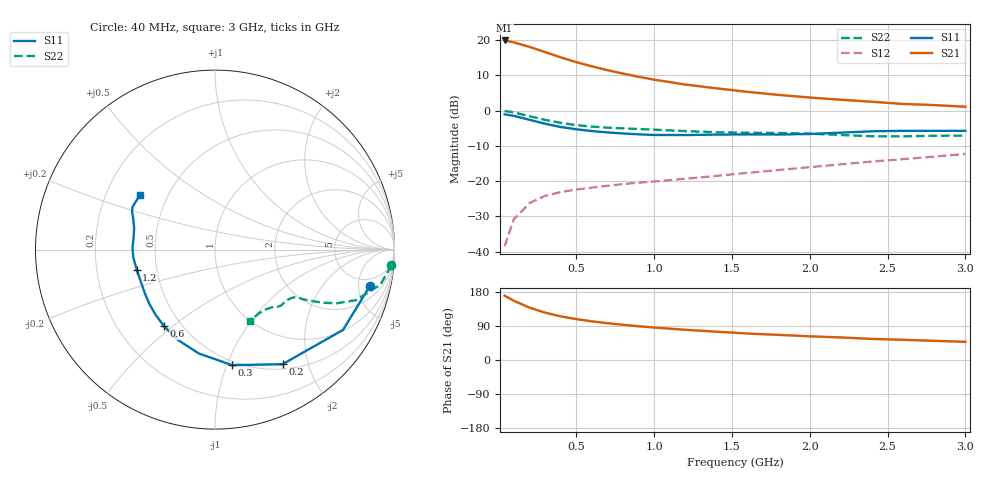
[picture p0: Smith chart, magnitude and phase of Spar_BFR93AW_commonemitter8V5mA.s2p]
! Filename:  BFR93AWE.S2P  Version:  4.0
! NXP part #: BFR93AW  Date: Jun 1994
! Bias condition: Vce=8V, Ic=5mA
#  MHz  S  MA  R  50
! Freq  S11  S21  S12  S22  !GUM [dB]
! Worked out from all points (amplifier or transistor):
!   21 points, 40 MHz to 3 GHz, reference 50 ohm
!   highest |S21| = 19.9 dB at 40 MHz (marker M1)
!   |S21| within 3 dB of that: start of sweep to 280.1 MHz
!   unconditionally stable (mu >= 1): 1.043 GHz to end of sweep
!   at 300 MHz: K = 0.40, MSG = 20.4 dB, |S12| = -24.2 dB
!   at 1 GHz: K = 0.98, MSG = 14.4 dB, |S12| = -20.1 dB
!   at 3 GHz: K = 1.05, MAG = 5.4 dB, |S12| = -12.3 dB
!   lowest NFmin = 1.20 dB at 500 MHz
!   S11 on the Smith chart (normalised r, x): 40 MHz: 3.55, -6.74; 200 MHz: 0.57, -1.60; 300 MHz: 0.47, -1.05; 600 MHz: 0.40, -0.47; 1.2 GHz: 0.38, -0.11; 3 GHz: 0.35, +0.29
40  0.886 -13.3  9.855 169.6  0.012 83.2  0.987 -5.1
100  0.842 -32.1  9.245 156.2  0.029 72.7  0.942 -12.0
200  0.741 -59.5  7.99 138.2  0.049 60.9  0.833 -19.8
300  0.651 -81.5  6.746 124.9  0.062 53.9  0.739 -23.9
400  0.586 -98.8  5.685 115.1  0.07 50.6  0.67 -26.2
500  0.544 -112.3  4.859 107.9  0.076 49.4  0.623 -27.6
600  0.513 -123.5  4.238 102.0  0.081 49.7  0.593 -28.5
700  0.491 -132.6  3.741 97.1  0.086 50.5  0.573 -29.1
800  0.474 -140.7  3.345 92.9  0.091 51.9  0.56 -29.5
900  0.461 -147.8  3.014 89.0  0.095 53.6  0.548 -29.7
1000  0.452 -154.3  2.745 85.7  0.099 55.2  0.537 -30.0
1200  0.45 -165.7  2.341 79.8  0.108 58.7  0.512 -31.3
1400  0.457 -174.3  2.068 74.7  0.119 62.1  0.494 -34.1
1600  0.46 178.9  1.843 69.9  0.131 65.0  0.485 -37.7
1800  0.458 172.3  1.667 66.3  0.144 68.1  0.482 -40.3
2000  0.466 165.2  1.531 62.5  0.158 70.5  0.472 -42.4
2200  0.487 159.3  1.425 59.5  0.173 72.6  0.451 -45.5
2400  0.509 155.2  1.333 55.6  0.19 74.1  0.433 -50.9
2600  0.517 152.7  1.242 53.3  0.205 75.0  0.432 -56.9
2800  0.516 148.7  1.196 50.6  0.223 76.2  0.44 -61.1
3000  0.517 143.9  1.134 48.0  0.243 76.9  0.441 -64.1
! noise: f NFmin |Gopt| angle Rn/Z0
500  1.2  0.313  45.9  0.163
1000  1.9  0.28  133.8  0.218
2000  3  0.606  -155.7  0.137
